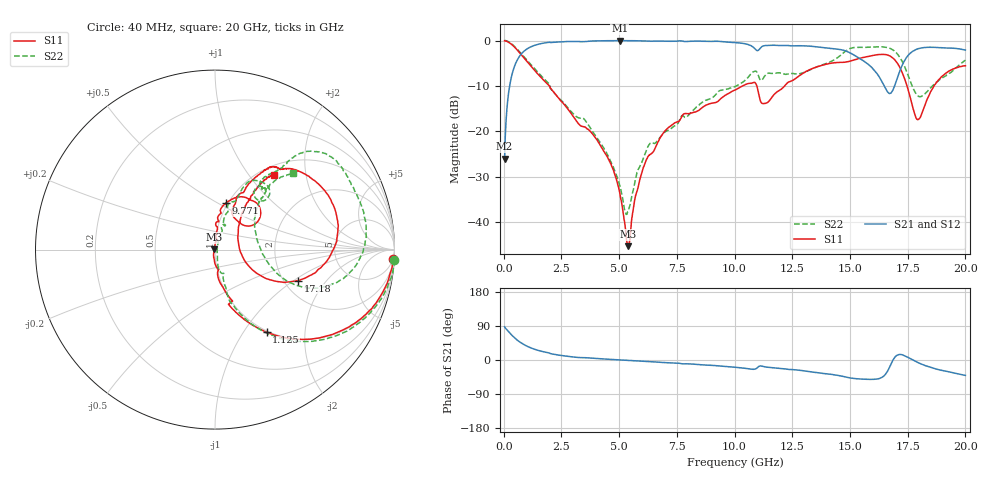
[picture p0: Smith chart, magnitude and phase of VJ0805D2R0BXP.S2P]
! VJ0805D2R0BXP
! DATE 10/29/2021  11:32
! CAPACITORS MOUNTED IN SERIES ON 25 MIL THICK MICROSTRIP SUBSTRATE
# GHz  S  MA  R  50.00
!  FREQ  S11M  S11A  S21M  S21A  S12M  S12A  S22M  S22A
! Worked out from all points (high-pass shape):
!   1601 points, 40 MHz to 20 GHz, reference 50 ohm
!   highest |S21| = -0.01 dB at 5.03 GHz (marker M1); lowest = -26.0 dB at 40 MHz (marker M2)
!   |S21| within 3 dB of the highest: 752.1 MHz to 15.11 GHz (14.36 GHz wide, 181 % of centre); 17.56 GHz to end of sweep
!   lowest |S11| = -45.2 dB at 5.392 GHz (marker M3), VSWR 1.01, Z = 49.5 + j0.0562 ohm
!   |S11| at or under -10 dB: 1.984 GHz to 10.34 GHz (8.356 GHz wide, 136 % of centre); 10.97 GHz to 12.17 GHz (1.2 GHz wide, 10.4 % of centre); 17.47 GHz to 18.64 GHz (1.169 GHz wide, 6.47 % of centre)
!   |S22| runs from -38.2 to 0.0 dB; largest |S21 - S12| = 0.0054
!   S11 on the Smith chart (normalised r, x): 40 MHz: 4, -37; 1.125 GHz: 0.98, -1.28; 9.771 GHz: 0.98, +0.54; 17.18 GHz: 2.39, -1.09; 20 GHz: 1.16, +1.33
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0.04  0.9941 -3.0  0.05026 87.7  0.05235 87.3  1 -3.3
0.202175  0.9623 -14.7  0.253 75.1  0.2533 75.3  0.9734 -14.8
0.376825  0.8929 -26.1  0.44 64.0  0.4399 63.9  0.9055 -26.4
1.125325  0.5424 -58.0  0.8413 33.3  0.8404 33.2  0.563 -57.2
3.370825  0.1144 -79.8  0.9717 6.2  0.9705 6.1  0.1406 -70.3
4.45615  0.05404 -94.9  0.9952 2.3  0.995 2.3  0.05773 -76.7
5.03  0.02091 -111.7  0.9987 0.2  0.9986 0.2  0.02539 -58.6
5.391775  0.005475 174.0  0.9968 -1.1  0.9962 -1.2  0.01317 15.0
5.990575  0.03549 87.1  0.9933 -3.4  0.9924 -3.4  0.04646 67.6
6.70165  0.07782 86.2  0.9877 -5.7  0.9863 -5.7  0.0815 68.0
9.7705  0.2645 77.0  0.9587 -17.9  0.9582 -18.1  0.2977 67.0
10.02  0.2856 73.1  0.9492 -19.1  0.9484 -19.2  0.3122 66.6
10.84335  0.3478 48.5  0.8319 -24.6  0.8317 -24.6  0.4572 55.7
11.34235  0.2039 54.9  0.8823 -18.4  0.8819 -18.5  0.4192 56.0
13.35083  0.4897 59.2  0.8646 -31.5  0.8628 -31.7  0.4865 55.8
14.93515  0.5872 49.8  0.7468 -46.5  0.7467 -46.6  0.803 42.5
15.93315  0.6812 32.7  0.5089 -51.2  0.5083 -51.2  0.8474 21.3
16.68165  0.6849 6.2  0.2638 -23.2  0.2636 -23.3  0.8282 0.6
17.18065  0.4959 -20.3  0.4796 14.6  0.4784 14.5  0.6403 -18.9
17.9541  0.1352 12.2  0.814 -7.1  0.8125 -7.2  0.2457 6.4
18.88972  0.3804 55.6  0.8357 -26.1  0.8354 -26.3  0.3726 47.1
20  0.5279 51.7  0.787 -40.6  0.7863 -40.8  0.6086 44.2
